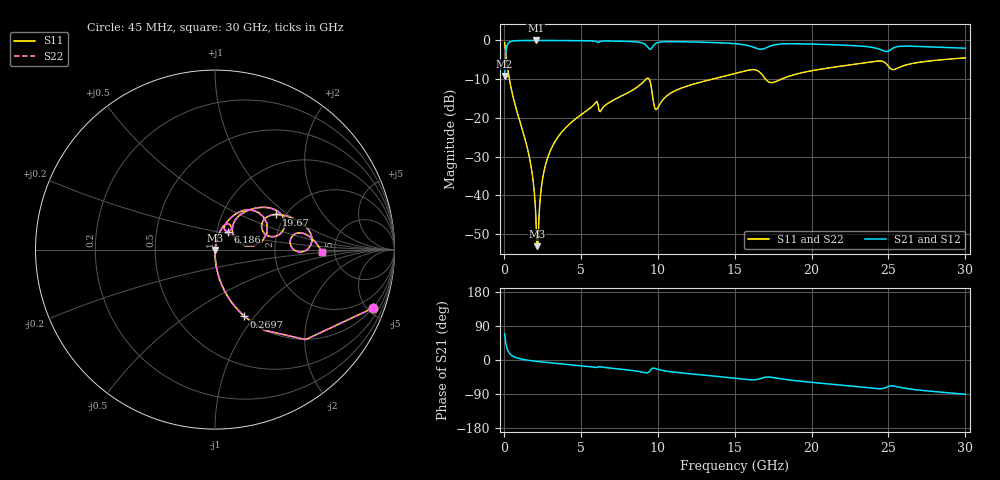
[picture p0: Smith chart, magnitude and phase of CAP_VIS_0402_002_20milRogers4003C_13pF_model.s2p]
! S-parameter model data by Modelithics Inc.  support@modelithics.com  813-866-6335  Tampa FL USA
! S-Parameter data specifications:
! Substrate: 20-mil Rogers 4003C, substrate thickness, H=0.508mm, Dielectric constant, Er=3.75
! PCB Mounting Pad Footprint: Pad width, PadW=0.50mm , Pad length, PadL=0.50mm , Pad gap, PadG (edge-to-edge)=0.40mm , Reference planes=1.4mm apart
! Created Wed Nov 18 12:51:44 2015
# hz S ma R 50
! 2 Port Network Data from SP1.SP block
! freq  magS11  angS11  magS21  angS21  magS12  angS12  magS22  angS22
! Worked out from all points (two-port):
!   401 points, 45 MHz to 30 GHz, reference 50 ohm
!   highest |S21| = -0.01 dB at 2.067 GHz (marker M1); lowest = -9.2 dB at 45 MHz (marker M2)
!   |S21| within 3 dB of the highest: 122.6 MHz to end of sweep
!   lowest |S11| = -53.1 dB at 2.142 GHz (marker M3), VSWR 1.00, Z = 50.1 - j0.19 ohm
!   |S11| at or under -10 dB: 356.4 MHz to 9.236 GHz (8.88 GHz wide, 185 % of centre); 9.435 GHz to 13.55 GHz (4.111 GHz wide, 35.8 % of centre); 17.02 GHz to 18.03 GHz (1.018 GHz wide, 5.81 % of centre)
!   |S22| runs from -53.1 to -0.6 dB; largest |S21 - S12| = 0
!   S11 on the Smith chart (normalised r, x): 45 MHz: 0.99, -5.40; 269.7 MHz: 0.99, -0.89; 6.186 GHz: 1.14, +0.23; 19.67 GHz: 1.79, +0.83; 30 GHz: 3.94, -0.15
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4.5e7  0.938 -20.3  0.3464 69.6  0.3464 69.6  0.938 -20.3
2.696625e8  0.4065 -66.4  0.9132 23.5  0.9132 23.5  0.4065 -66.4
5.692125e8  0.1956 -79.5  0.98 10.3  0.98 10.3  0.1956 -79.5
1.692525e9  0.02858 -89.0  0.9984 -1.3  0.9984 -1.3  0.02858 -89.0
2.066962e9  0.005958 -81.2  0.9987 -3.3  0.9987 -3.3  0.005958 -81.2
2.14185e9  0.002216 -58.8  0.9987 -3.6  0.9987 -3.6  0.002216 -58.8
2.291625e9  0.00595 73.0  0.9986 -4.3  0.9986 -4.3  0.00595 73.0
2.591175e9  0.01984 80.3  0.9983 -5.6  0.9983 -5.6  0.01984 80.3
3.0405e9  0.03864 80.2  0.9976 -7.5  0.9976 -7.5  0.03864 80.2
5.062462e9  0.1117 73.6  0.9912 -15.2  0.9912 -15.2  0.1117 73.6
6.185775e9  0.1231 53.1  0.9521 -17.4  0.9521 -17.4  0.1231 53.1
9.33105e9  0.3257 34.1  0.8307 -33.8  0.8307 -33.8  0.3257 34.1
9.855262e9  0.1287 26.2  0.9104 -22.7  0.9104 -22.7  0.1287 26.2
1.007992e10  0.1437 47.5  0.9481 -25.4  0.9481 -25.4  0.1437 47.5
1.135301e10  0.2348 54.4  0.9626 -33.3  0.9626 -33.3  0.2348 54.4
1.50225e10  0.3736 38.8  0.9074 -48.1  0.9074 -48.1  0.3736 38.8
1.696958e10  0.3243 12.8  0.7908 -45.7  0.7908 -45.7  0.3243 12.8
1.966552e10  0.394 29.8  0.9006 -57.6  0.9006 -57.6  0.394 29.8
2.003996e10  0.4072 28.6  0.8967 -59.1  0.8967 -59.1  0.4072 28.6
2.438344e10  0.5433 7.3  0.7745 -75.7  0.7745 -75.7  0.5433 7.3
2.505742e10  0.4483 -0.9  0.7407 -68.9  0.7407 -68.9  0.4483 -0.9
3e10  0.5956 -1.2  0.7933 -90.3  0.7933 -90.3  0.5956 -1.2
